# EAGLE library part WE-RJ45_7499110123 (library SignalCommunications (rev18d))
Order Code 7499110123 Design THT xBase-T 10/100/1000 Base-T Ports 1x1 Application Standard Tab Position VERTICAL LED (Left-Right) YELLOW-GREEN EMI Fingers No Details see: http://katalog.we-online.de/en/pbs/WE-LAN_RJ45/7499110123? Updated by Yingchun Shan 2016-08-29 2016(C) Würth Elektronik
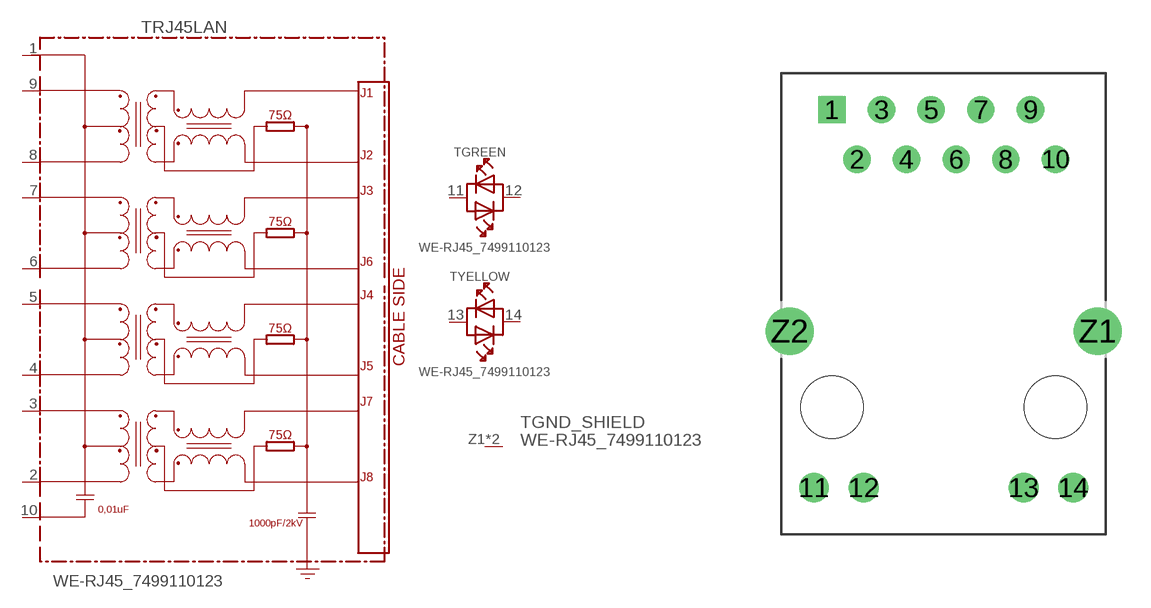
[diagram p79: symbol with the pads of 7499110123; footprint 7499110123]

Designator prefix T; gates RJ45LAN=7499110123 GND_SHIELD=GNDPIN GREEN=LED-DUAL YELLOW=LED-DUAL

## WE-RJ45_7499110123 (COMPANY-URL: http://www.we-online.de; CREATED-BY: Christin Zierenner; CREATED-DATE: AUG 2012; DATASHEET-URL: http://katalog.we-online.de/kataloge/eisos/media/pdf/7499110123.pdf; MANUFACTURER: Würth Elektronik eiSos GmbH)  [7499110123]
1  RJ45LAN:1
2  RJ45LAN:9
3  RJ45LAN:8
4  RJ45LAN:7
5  RJ45LAN:6
6  RJ45LAN:5
7  RJ45LAN:4
8  RJ45LAN:3
9  RJ45LAN:2
10  RJ45LAN:10
11  GREEN:AK1  pas
12  GREEN:AK2  pas
13  YELLOW:AK1  pas
14  YELLOW:AK2  pas
Z1  GND_SHIELD:GND  pwr
Z2  GND_SHIELD:GND  pwr

## Footprint 7499110123 (pad centres in mm)
MAX HEIGHT=17.10mm PORTS----1X1 LED -YES
drill 0.89 square: 1 -5.72,15.24
drill 0.89: 2 -4.44,12.7; 3 -3.18,15.24; 4 -1.9,12.7; 5 -0.64,15.24; 6 0.64,12.7; 7 1.9,15.24; 8 3.18,12.7; 9 4.44,15.24; 10 5.72,12.7
drill 1.02: 11 -6.635,-4.11; 12 -4.095,-4.11; 13 4.095,-4.11; 14 6.635,-4.11
drill 1.63: Z1 7.875,3.89; Z2 -7.875,3.89
hole 3.2 at -5.715,0
hole 3.2 at 5.715,0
